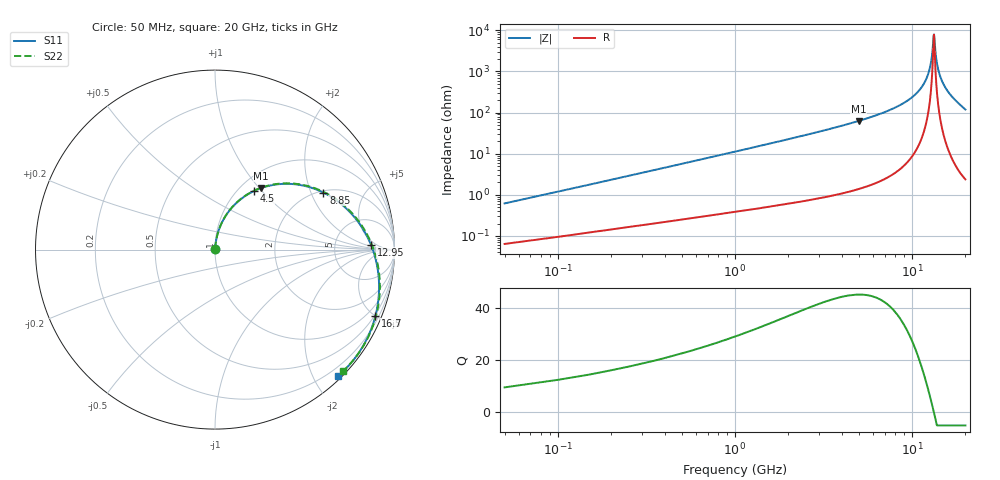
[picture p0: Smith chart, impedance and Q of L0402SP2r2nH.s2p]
!	AVX Thin Film Operation
!	Date:		5 January 2004
!	Description: 	Accu-L®  L0402 Series Thin Film RF Inductors
!	Part Number:	L04022R2AHLTR
!	50 MHz-20GHz Serial Measurements
#	mhz	S	db	R	50
!	S11	S11	S21	S21	S12	S12	S22	S22
!	dB	Phase	dB	Phase	dB	Phase	dB	Phase
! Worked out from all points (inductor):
!   400 points, 50 MHz to 20 GHz, reference 50 ohm
!   read as 1/Y11, port 2 shorted: L = 1.85 nH near 150 MHz
!   highest Q = 45.2 at 5 GHz (marker M1), where L = 1.99 nH
!   self-resonance near 13.25 GHz
!   S11 on the Smith chart (normalised r, x): 50 MHz: 1.00, +0.01; 4.5 GHz: 1.17, +0.90; 8.85 GHz: 2.07, +2.47; 12.95 GHz: 14, +3; 16.7 GHz: 0.44, -5.01; 20 GHz: 0.06, -2.37
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50  -45.49 82.7  -0.01 -0.4  -0.01 -0.4  -45.49 82.7
100  -39.84 83.9  -0.01 -0.8  -0.01 -0.8  -39.84 83.9
150  -36.49 84.2  -0.01 -1.2  -0.01 -1.2  -36.49 84.2
250  -32.24 84.3  -0.02 -1.9  -0.02 -1.9  -32.24 84.3
450  -27.32 83.5  -0.03 -3.4  -0.03 -3.4  -27.32 83.5
800  -22.48 81.6  -0.05 -5.9  -0.05 -5.9  -22.48 81.6
1800  -15.66 75.0  -0.17 -13.1  -0.17 -13.1  -15.66 75.1
3400  -10.40 64.0  -0.49 -24.4  -0.49 -24.4  -10.40 64.2
4500  -8.17 56.5  -0.81 -32.0  -0.81 -32.0  -8.17 56.8
5000  -7.36 53.1  -0.98 -35.4  -0.98 -35.4  -7.36 53.4
6700  -5.19 41.7  -1.69 -46.8  -1.69 -46.8  -5.19 42.2
8850  -3.32 27.7  -2.90 -60.7  -2.90 -60.7  -3.32 28.3
10050  -2.54 20.0  -3.76 -68.3  -3.76 -68.3  -2.54 20.7
12950  -1.21 1.7  -6.56 -86.2  -6.56 -86.2  -1.21 2.6
13350  -1.08 -0.8  -7.06 -88.6  -7.06 -88.6  -1.08 0.2
16700  -0.29 -22.4  -13.97 -108.2  -13.97 -108.2  -0.29 -21.0
18250  -0.14 -33.0  -22.66 -112.2  -22.66 -112.2  -0.13 -31.3
18650  -0.12 -35.8  -27.96 -106.2  -27.96 -106.2  -0.12 -34.1
19050  -0.12 -38.7  -37.58 -48.6  -37.58 -48.6  -0.11 -36.8
19150  -0.12 -39.4  -36.75 -12.0  -36.75 -12.0  -0.11 -37.5
19550  -0.13 -42.3  -26.96 31.5  -26.96 31.5  -0.12 -40.4
20000  -0.15 -45.7  -21.33 36.3  -21.33 36.3  -0.15 -43.6
